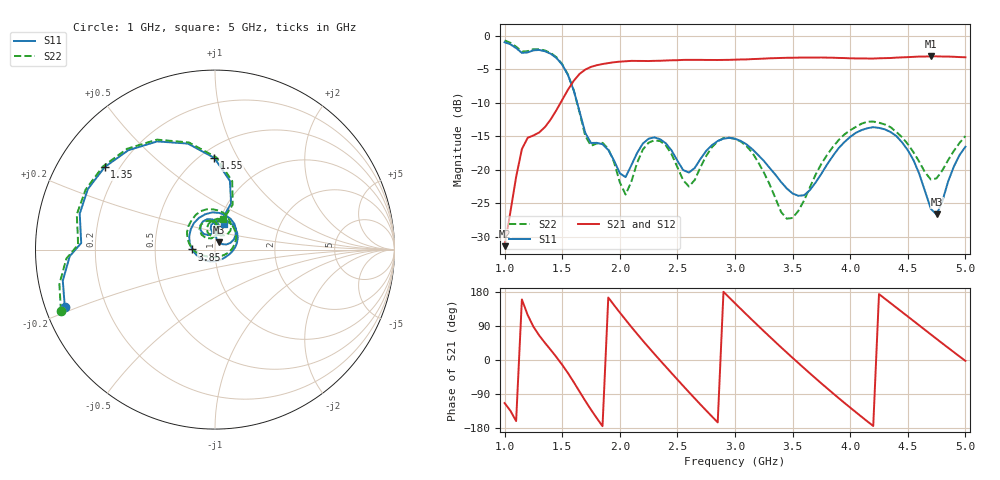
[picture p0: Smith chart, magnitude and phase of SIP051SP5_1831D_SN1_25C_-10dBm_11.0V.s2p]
# GHz  S  dB  R  50
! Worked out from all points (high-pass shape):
!   81 points, 1 GHz to 5 GHz, reference 50 ohm
!   highest |S21| = -3.06 dB at 4.7 GHz (marker M1); lowest = -31.4 dB at 1 GHz (marker M2)
!   |S21| within 3 dB of the highest: 1.632 GHz to end of sweep
!   lowest |S11| = -26.7 dB at 4.75 GHz (marker M3), VSWR 1.10, Z = 52.1 + j4.24 ohm
!   |S11| at or under -10 dB: 1.63 GHz to end of sweep
!   |S22| runs from -27.3 to -0.7 dB; largest |S21 - S12| = 0.0027
!   S11 on the Smith chart (normalised r, x): 1 GHz: 0.06, -0.18; 1.35 GHz: 0.15, +0.33; 1.55 GHz: 0.58, +0.81; 3.85 GHz: 0.77, +0.00; 5 GHz: 1.06, +0.30
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1  -0.95 -159.1  -31.40 -113.6  -31.34 -114.5  -0.69 -158.3
1.15  -2.54 177.2  -16.91 159.8  -16.92 159.9  -2.34 178.0
1.35  -2.29 143.2  -13.62 45.3  -13.62 45.3  -2.18 143.5
1.55  -5.84 90.4  -8.04 -34.6  -8.02 -34.6  -5.79 89.1
1.7  -14.46 75.3  -5.03 -107.7  -5.03 -107.6  -14.92 74.2
1.85  -16.17 93.3  -4.21 -174.6  -4.20 -174.6  -15.97 92.3
2.05  -21.09 114.4  -3.79 106.2  -3.81 106.2  -23.68 107.1
2.2  -16.07 121.4  -3.75 51.0  -3.74 51.1  -16.97 127.5
2.35  -15.43 95.4  -3.72 -1.0  -3.71 -1.0  -15.71 98.4
2.5  -18.64 79.7  -3.63 -51.6  -3.63 -51.6  -19.61 77.9
2.65  -19.73 99.7  -3.58 -101.1  -3.58 -101.1  -21.53 107.8
2.85  -15.69 84.1  -3.60 -164.6  -3.61 -164.5  -15.74 95.2
3  -15.36 56.3  -3.56 149.8  -3.55 149.9  -15.39 63.2
3.3  -19.70 -0.2  -3.35 61.9  -3.35 61.9  -22.15 -11.4
3.5  -23.53 -49.2  -3.27 5.7  -3.26 5.6  -27.18 -99.2
3.7  -21.89 -130.7  -3.24 -48.6  -3.23 -48.5  -20.71 -164.9
3.85  -17.92 179.7  -3.26 -87.8  -3.26 -87.7  -16.57 166.5
4.1  -14.06 116.6  -3.37 -150.1  -3.36 -150.1  -13.10 118.9
4.35  -14.36 62.6  -3.31 150.3  -3.31 150.3  -13.63 75.5
4.7  -25.83 36.4  -3.06 67.4  -3.05 67.5  -21.44 68.5
4.75  -26.66 60.9  -3.06 55.7  -3.07 55.6  -21.27 80.1
5  -16.56 70.7  -3.20 -2.2  -3.20 -2.0  -14.96 75.0
